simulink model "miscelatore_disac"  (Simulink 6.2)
settings: Solver=ode15s  StartTime=0.0  StopTime=5000  RelTol=1e-3
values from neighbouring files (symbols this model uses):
  A = pi    (= 3.14159265359)    [dati_miscelatore.m]
  c = 4200    [dati_miscelatore.m]
  k = 0.36    [dati_miscelatore.m]
  R = ((c*w1+c*w2+k*A)*T-c*w1*T1-c*w2*T2-k*A*Ta)/(i^2)    (= 7560)    [dati_miscelatore.m]
  rho = 1000    [dati_miscelatore.m]
  T1 = 273+50    (= 323)    [dati_miscelatore.m]
  T2 = 273+10    (= 283)    [dati_miscelatore.m]
  Ta = 273+20    (= 293)    [dati_miscelatore.m]
undefined symbols (not defined in the file or in its folder): miscelatore

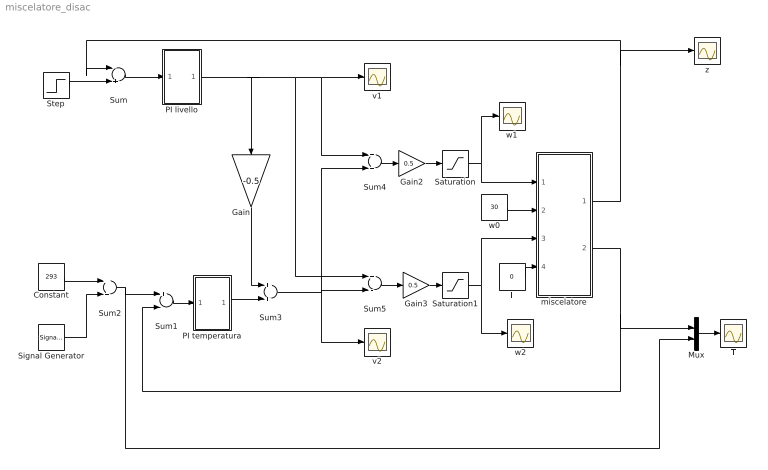
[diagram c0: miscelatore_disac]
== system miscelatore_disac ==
  Constant : Constant  Value=293
  Gain : Gain  Orientation=down  Gain=-0.5
  Gain2 : Gain  Gain=0.5
  Gain3 : Gain  Gain=0.5
  Mux : Mux  Inputs=2
  PI livello : Subsystem
  PI temperatura : Subsystem
  Saturation : Saturate  UpperLimit=20  LowerLimit=0
  Saturation1 : Saturate  UpperLimit=40  LowerLimit=15
  Signal Generator : SignalGenerator  WaveForm=square  Amplitude=5  Frequency=.0005
  Step : Step  Time=0  Before=1  SampleTime=0
  Sum : Sum  Inputs=-+
  Sum1 : Sum  Inputs=+-
  Sum2 : Sum
  Sum3 : Sum
  Sum4 : Sum
  Sum5 : Sum  Inputs=+-
  T : Scope
  i : Constant  Value=0
  miscelatore : Subsystem
  v1 : Scope
  v2 : Scope
  w0 : Constant  Value=30
  w1 : Scope
  w2 : Scope
  z : Scope
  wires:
  miscelatore/1(Out1) -> Sum/1, z/1
  miscelatore/2(Out2) -> Sum1/2, Mux/1
  Step/1 -> Sum/2
  Sum1/1 -> PI temperatura/1(In1)
  Sum2/1 -> Sum1/1, Mux/2
  Constant/1 -> Sum2/1
  Signal Generator/1 -> Sum2/2
  i/1 -> miscelatore/4(In4)
  w0/1 -> miscelatore/2(In2)
  PI temperatura/1(Out1) -> Sum3/2
  Gain/1 -> Sum3/1
  PI livello/1(Out1) -> Gain/1, Sum5/1, Sum4/1, v1/1
  Sum3/1 -> Sum4/2, Sum5/2, v2/1
  Sum/1 -> PI livello/1(In1)
  Sum4/1 -> Gain2/1
  Sum5/1 -> Gain3/1
  Mux/1 -> T/1
  Gain2/1 -> Saturation/1
  Saturation/1 -> miscelatore/1(In1), w1/1
  Gain3/1 -> Saturation1/1
  Saturation1/1 -> miscelatore/3(In3), w2/1

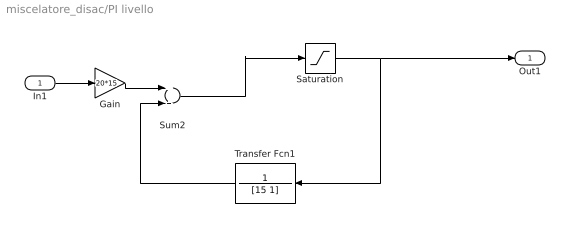
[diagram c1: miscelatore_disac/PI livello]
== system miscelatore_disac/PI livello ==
  In1 : Inport  Port=1  LatchInput=off
  Gain : Gain  Gain=20*15
  Saturation : Saturate  UpperLimit=60  LowerLimit=15
  Sum2 : Sum
  Transfer Fcn1 : TransferFcn  Orientation=left  Numerator=1  Denominator=[15 1]
  Out1 : Outport
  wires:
  Gain/1 -> Sum2/1
  Transfer Fcn1/1 -> Sum2/2
  In1/1 -> Gain/1
  Saturation/1 -> Transfer Fcn1/1, Out1/1
  Sum2/1 -> Saturation/1

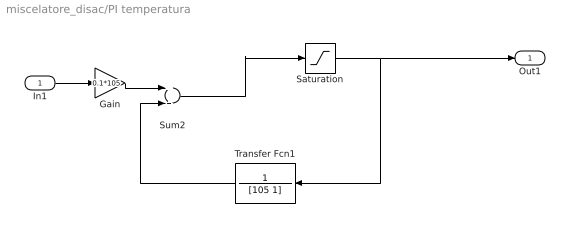
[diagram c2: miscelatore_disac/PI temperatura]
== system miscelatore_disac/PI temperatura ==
  In1 : Inport  Port=1  LatchInput=off
  Gain : Gain  Gain=0.1*105
  Saturation : Saturate  UpperLimit=40  LowerLimit=-40
  Sum2 : Sum
  Transfer Fcn1 : TransferFcn  Orientation=left  Numerator=1  Denominator=[105 1]
  Out1 : Outport
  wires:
  Gain/1 -> Sum2/1
  Transfer Fcn1/1 -> Sum2/2
  In1/1 -> Gain/1
  Saturation/1 -> Transfer Fcn1/1, Out1/1
  Sum2/1 -> Saturation/1

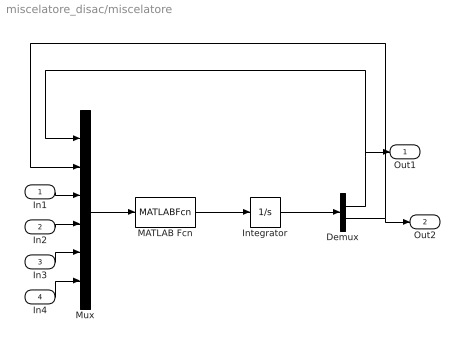
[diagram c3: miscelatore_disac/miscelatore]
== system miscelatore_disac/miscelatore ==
  In1 : Inport  Port=1  LatchInput=off
  In2 : Inport  Port=2  LatchInput=off
  In3 : Inport  Port=3  LatchInput=off
  In4 : Inport  Port=4  LatchInput=off
  Demux : Demux  Outputs=2
  Integrator : Integrator  InitialCondition=[1 273+20]
  MATLAB Fcn : MATLABFcn  MATLABFcn=miscelatore(u,rho,A,c,T1,T2,Ta,k,R)
  Mux : Mux  Inputs=6
  Out1 : Outport
  Out2 : Outport  Port=2
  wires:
  Mux/1 -> MATLAB Fcn/1
  Demux/1 -> Mux/1, Out1/1
  Demux/2 -> Mux/2, Out2/1
  MATLAB Fcn/1 -> Integrator/1
  Integrator/1 -> Demux/1
  In1/1 -> Mux/3
  In2/1 -> Mux/4
  In3/1 -> Mux/5
  In4/1 -> Mux/6
